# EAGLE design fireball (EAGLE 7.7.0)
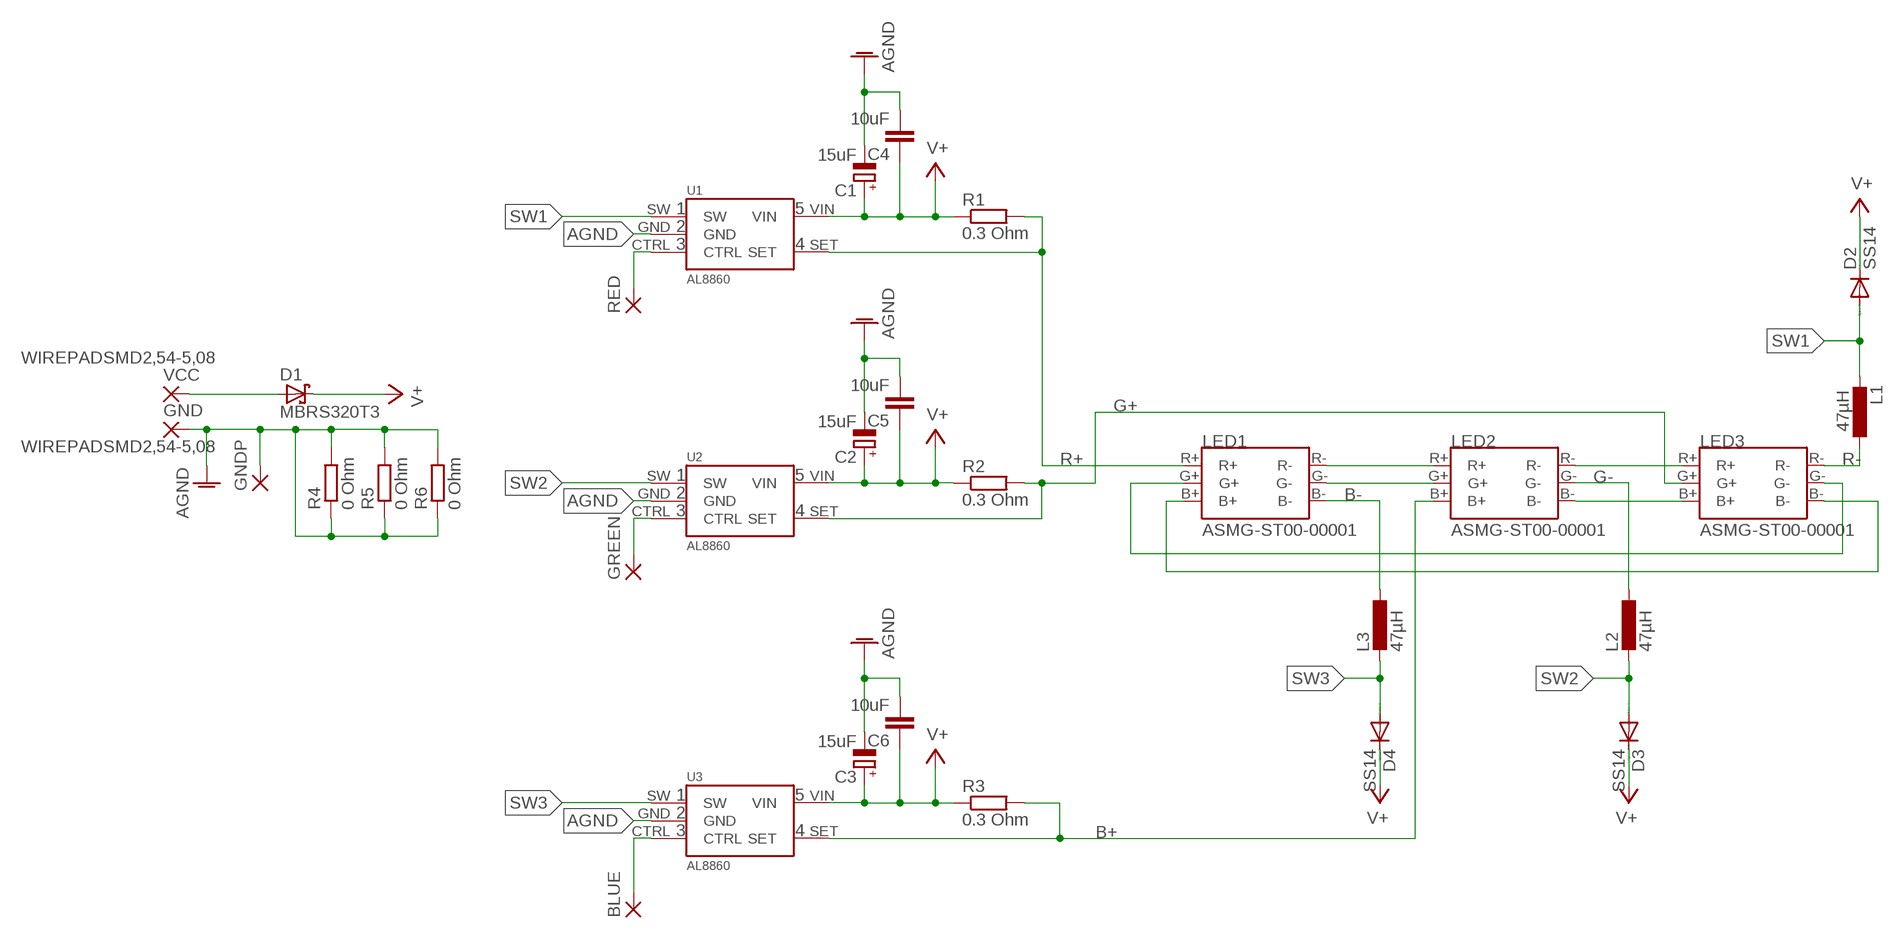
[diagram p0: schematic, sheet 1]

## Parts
BLUE  SMD2  [SMD1,27-2,54]
C1  15uF  CPOL-EUD/7343-31R  [D/7343-31R]
C2  15uF  CPOL-EUD/7343-31R  [D/7343-31R]
C3  15uF  CPOL-EUD/7343-31R  [D/7343-31R]
C4  10uF  C-EUC0805  [C0805]
C5  10uF  C-EUC0805  [C0805]
C6  10uF  C-EUC0805  [C0805]
D1  MBRS320T3  [SMC]
D2  SS14  DIODE-DO-214AC  [DO-214AC]
D3  SS14  DIODE-DO-214AC  [DO-214AC]
D4  SS14  DIODE-DO-214AC  [DO-214AC]
GND  WIREPADSMD2,54-5,08  [SMD2,54-5,08]
GNDP  SMD2  [SMD1,27-2,54]
GREEN  SMD2  [SMD1,27-2,54]
L1  47µH  L-EUL5038P  [L5038P]
L2  47µH  L-EUL5038P  [L5038P]
L3  47µH  L-EUL5038P  [L5038P]
LED1  ASMG-ST00-00001  [SMD]
LED2  ASMG-ST00-00001  [SMD]
LED3  ASMG-ST00-00001  [SMD]
R1  0.3 Ohm  R-EU_R1210  [R1210]
R2  0.3 Ohm  R-EU_R1210  [R1210]
R3  0.3 Ohm  R-EU_R1210  [R1210]
R4  0 Ohm  R-EU_R1206  [R1206]
R5  0 Ohm  R-EU_R1206  [R1206]
R6  0 Ohm  R-EU_R1206  [R1206]
RED  SMD2  [SMD1,27-2,54]
U1  AL8860  [TSOT-25-5]
U2  AL8860  [TSOT-25-5]
U3  AL8860  [TSOT-25-5]
VCC  WIREPADSMD2,54-5,08  [SMD2,54-5,08]

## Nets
AGND: C1.- C2.- C3.- C4.2 C5.2 C6.2 GND.1(P) GNDP.1(P) R4.1 R4.2 R5.1 R5.2 R6.1 R6.2 U1.GND U2.GND U3.GND
B+: LED2.B+ R3.2 U3.SET
B-: L3.1 LED1.B-
G+: LED3.G+ R2.2 U2.SET
G-: L2.1 LED2.G-
N$2: LED2.B- LED3.B+
N$3: LED1.B+ LED3.B-
N$6: LED1.G- LED2.G+
N$7: LED1.G+ LED3.G-
N$11: LED1.R- LED2.R+
N$12: LED2.R- LED3.R+
N$13: GREEN.1(P) U2.CTRL
N$14: BLUE.1(P) U3.CTRL
N$15: RED.1(P) U1.CTRL
N$16: D1.A VCC.1(P)
R+: LED1.R+ R1.2 U1.SET
R-: L1.1 LED3.R-
SW1: D2.A L1.2 U1.SW
SW2: D3.A L2.2 U2.SW
SW3: D4.A L3.2 U3.SW
V+: C1.+ C2.+ C3.+ C4.1 C5.1 C6.1 D1.C D2.C D3.C D4.C R1.1 R2.1 R3.1 U1.VIN U2.VIN U3.VIN

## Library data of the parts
BLUE GNDP GREEN RED = wirepad:SMD2: SMD PAD
C1-C3 = rcl:CPOL-EU: POLARIZED CAPACITOR, European symbol
C4-C6 = rcl:C-EU: CAPACITOR, European symbol
D1 = diode:MBRS3*0T3: SCHOTTKY BARRIER RECTIFIER 3.0 AMPERES 20, 30, 40 VOLT
D2-D4 = diode:DIODE-: DIODE
GND VCC = wirepad:WIREPAD: Wire PAD connect wire on PCB
L1-L3 = rcl:L-EU: INDUCTOR, European symbol
LED1-LED3 = broadcom:ASMG-ST00-00001
R1-R6 = rcl:R-EU_: RESISTOR, European symbol
U1-U3 = AL8860WT:AL8860

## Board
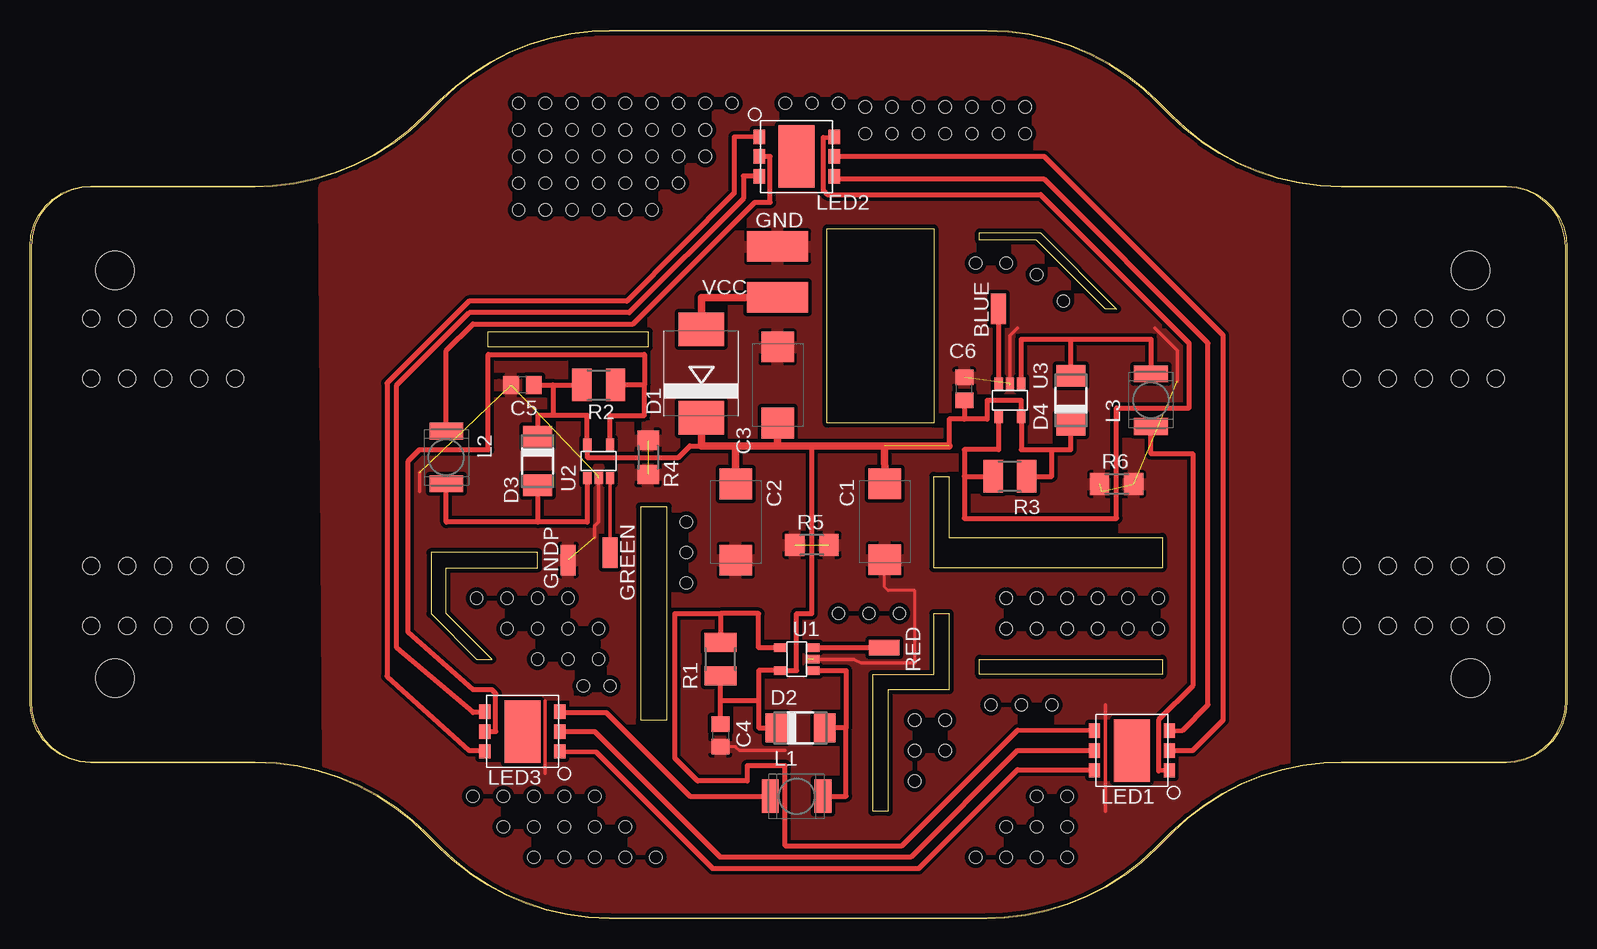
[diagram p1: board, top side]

Size 128.1 x 74.1 mm. Coordinates in mm from the lower left corner, seen from the top.
Outline: 551 segments
Copper layers (1*16): Top 0.035559375mm / dielectric 1.6mm / Bottom 0.035559375mm
Design rules "oshpark-2layer": minimum track width 6mil, minimum drill 10mil, track to track 6mil, track to pad 6mil, pad to pad 6mil, via to via 6mil, smd to smd 6mil, copper to edge 15mil, drill to drill 6mil, minimum pad ring 5mil, minimum via ring 5mil, stop-mask expansion 2.5mil, vias tented up to drill 0mil, thermal gap 10mil
Holes 3.2 mm at 120.09,20.05 120.09,54.05 7.09,54.05 7.09,20.05
Holes 1 mm at 42.32,21.64 44.86,21.64 47.4,21.64 47.4,24.18 44.86,26.72 44.86,24.18 42.32,24.18 42.32,26.72 39.78,26.72 39.78,24.18 37.24,26.72 83.91,26.72 86.45,26.72 88.99,26.72 91.53,26.72 83.91,24.18 86.45,24.18 88.99,24.18 91.53,24.18 81.37,26.72 81.37,24.18 94.07,26.72 94.07,24.18 73.75,16.56 76.29,16.56 73.75,14.02 76.29,14.02 73.75,11.48 83.91,10.21 86.45,10.21 86.45,7.67 83.91,7.67 81.37,7.67 78.83,5.13 81.37,5.13 83.91,5.13 86.45,5.13 67.4,25.45 69.94,25.45 72.48,25.45 54.7,33.07 54.7,30.53 54.7,27.99 47.08,10.21 44.54,10.21 44.54,7.67 42,10.21 39.46,10.21 36.92,10.21 39.46,7.67 42,7.67 47.08,7.67 47.08,5.13 44.54,5.13 42,5.13 49.62,5.13 49.62,7.67 52.16,5.13 78.83,54.66 81.37,54.66 83.91,53.71 86.14,51.48 80.1,17.83 82.64,17.83 85.18,17.83 69.62,65.45 71.85,65.45 74.07,65.45 76.29,65.45 78.52,65.45 80.74,65.45 82.96,65.45 69.62,67.68 71.85,67.68 74.07,67.68 76.29,67.68 78.52,67.68 80.74,67.68 82.96,67.68 58.51,67.99 62.96,67.99 67.4,67.99 65.18,67.99 46.13,19.42 48.35,19.42 56.29,67.99 54.07,67.99 51.84,67.99 49.62,67.99 56.29,65.77 56.29,63.55 54.07,65.77 54.07,63.55 51.84,61.33 51.84,63.55 51.84,65.77 49.62,65.77 49.62,63.55 49.62,61.33 47.4,67.99 45.18,67.99 42.95,67.99 40.73,67.99 40.73,65.77 42.95,65.77 45.18,65.77 47.4,65.77 47.4,63.55 45.18,63.55 42.95,63.55 40.73,63.55 40.73,61.33 42.95,61.33 45.18,61.33 47.4,61.33 40.73,59.1 42.95,59.1 45.18,59.1 47.4,59.1 49.62,59.1 51.84,59.1 54.07,61.33
Holes 1.4 mm at 5.09,50.05 8.09,50.05 11.09,50.05 14.09,50.05 17.09,50.05 5.09,45.05 8.09,45.05 11.09,45.05 14.09,45.05 17.09,45.05 5.09,29.41 8.09,29.41 11.09,29.41 14.09,29.41 17.09,29.41 5.09,24.41 8.09,24.41 11.09,24.41 14.09,24.41 17.09,24.41 110.19,50.05 113.19,50.05 116.19,50.05 119.19,50.05 122.19,50.05 110.19,45.05 113.19,45.05 116.19,45.05 119.19,45.05 122.19,45.05 110.19,29.41 113.19,29.41 116.19,29.41 119.19,29.41 122.19,29.41 110.19,24.41 113.19,24.41 116.19,24.41 119.19,24.41 122.19,24.41

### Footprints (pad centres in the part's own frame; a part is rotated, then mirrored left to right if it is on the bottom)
SMD1,27-2,54 = smd 1.27 x 2.54: 1 0,0
D/7343-31R = smd 2.55 x 2.7: + 3.175,0; - -3.175,0
C0805 = smd 1.3 x 1.5: 1 -0.95,0; 2 0.95,0
SMC = smd 2.8 x 3.8: A 3.7,0; C -3.7,0
DO-214AC = smd 1.8 x 2.4: A 2.025,0; C -2.025,0
SMD2,54-5,08 = smd 2.54 x 5.08: 1 0,0
L5038P = smd 1.4 x 2.8: 1 -2.2,0; 2 2.2,0
SMD = smd 0.95 x 1.2: B+ -3.125,-1.65; B- 3.125,-1.65; G+ -3.125,0; G- 3.125,0; R+ -3.125,1.65; R- 3.125,1.65 | smd 3 x 5.2: NC 0,0
R1210 = smd 1.6 x 2.7: 1 -1.4,0; 2 1.4,0
R1206 = smd 1.6 x 1.803: 1 -1.422,0; 2 1.422,0
TSOT-25-5 = smd 1 x 0.7: CTRL -1.4,-0.95; GND -1.4,0; SET 1.4,-0.95; SW -1.4,0.95; VIN 1.4,0.95

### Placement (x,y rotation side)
BLUE  80.74,50.85 0 top
C1  71.25,33.09 90 top
C2  58.83,33.07 90 top
C3  62.32,44.5 270 top
C4  57.56,15.29 270 top
C5  41.05,44.5 180 top
C6  77.88,44.18 90 top
D1  55.97,45.45 90 top
D2  64.23,15.93 0 top
D3  42.32,38.15 270 top
D4  86.77,43.23 90 top
GND  62.31,56.05 90 top
GNDP  44.86,29.89 0 top
GREEN  48.35,30.53 180 top
L1  63.91,10.21 0 top
L2  34.7,38.47 270 top
L3  93.44,43.23 90 top
LED1  91.85,14.02 0 top
LED2  63.91,63.55 180 top
LED3  41.05,15.61 0 top
R1  57.56,21.64 90 top
R2  47.4,44.5 0 top
R3  81.69,36.88 180 top
R4  51.53,38.47 90 top
R5  65.18,31.16 0 top
R6  90.58,36.24 0 top
RED  71.21,22.59 90 top
U1  63.91,21.64 180 top
U2  47.4,38.15 90 top
U3  81.69,43.23 270 top
VCC  62.32,51.8 270 top

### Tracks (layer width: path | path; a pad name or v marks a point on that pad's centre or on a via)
AGND  (12 unrouted)
  Top 0.254: 59.15,14.02 58.83,14.34 C4.2 | 68.67,21.64 69.31,21.32 | 73.75,21.32 73.75,27.36 71.53,27.36 71.21,27.67 71.21,30.21
  Top 0.305: 89.63,17.83 89.63,8.94 | 42.95,18.15 42.95,12.12 | 81.69,44.5 81.69,48.63 82.33,49.26 | 64.86,21.64 68.67,21.64 | 62.96,14.02 59.15,14.02 | 69.31,21.32 73.75,21.32 | 47.4,36.88 47.4,33.07 47.08,32.75 47.08,31.8 | 32.48,37.2 32.48,35.61 | 93.75,49.26 95.66,47.36 95.66,44.82
  Top 0.406: 89.31,35.61 89.31,36.88
  pour Top (isolate 0.305): 42.32,73.71 85.5,73.71 104.55,61.01 104.55,12.75 86.77,0.05 42.32,0.05 24.86,12.75 24.54,61.01
B+
  Top 0.406: U3.SET 80.74,39.1 77.88,39.1 77.88,36.88 | 77.88,36.88 77.88,33.39 90.58,33.39 90.58,42.59 96.61,42.59 96.61,47.99 84.23,60.38 66.45,60.38 66.13,60.69 66.13,65.14 LED2.B+ | 77.88,36.88 R3.2
B-
  Top 0.406: L3.1 93.44,38.78 96.93,38.78 96.93,19.42 94.07,16.56 94.07,12.32 LED1.B-
G+
  Top 0.406: U2.SET 48.35,40.69 48.35,41.96 51.21,41.96 51.21,44.5 | LED3.G+ 38.83,15.61 38.83,18.78 38.51,19.1 36.92,19.1 31.53,23.86 31.53,38.15 32.48,39.1 38.19,39.1 38.19,47.04 51.21,47.04 51.21,44.5 | 51.21,44.5 R2.2
G-
  Top 0.406: LED2.G- 61.69,63.55 61.69,59.74 60.42,59.74 50.26,49.58 36.92,49.58 34.7,47.36 L2.1
N$2
  Top 0.406: 37.8,14.02 LED3.B+ 37.69,14.02 36.61,14.02 29.76,20.21 29.76,44.65 36.59,51.48 49.76,51.48 58.69,60.49 58.69,65.17 LED2.B-
N$3
  Top 0.406: LED1.B+ 88.6,12.43 82.33,12.43 74.07,4.18 56.93,4.18 47.19,13.91 LED3.B-
N$6
  Top 0.406: LED1.G- 96.93,14.02 99.47,16.56 99.47,48.63 84.55,63.55 LED2.G+
N$7
  Top 0.406: LED1.G+ 82.33,14.02 73.44,5.13 57.56,5.13 47.08,15.61 LED3.G-
N$11
  Top 0.406: LED1.R- 96.09,15.72 98.2,17.83 98.2,47.99 84.55,61.64 67.36,61.64 LED2.R+
N$12
  Top 0.406: LED3.R+ 37.8,17.2 36.92,17.2 30.57,22.59 30.57,44.5 36.61,50.53 49.94,50.53 59.47,60.06 59.47,61.93 LED2.R-
N$13
  Top 0.305: GREEN.1 U2.CTRL
  Top 0.406: U2.CTRL
N$14
  Top 0.406: BLUE.1 80.74,48.31 U3.CTRL
N$15
  Top 0.406: RED.1 68.36,22.59 U1.CTRL
N$16
  Top 0.61: VCC.1 55.97,51.8 D1.A
R+
  Top 0.406: 57.56,25.45 R1.2 | U1.SET 60.73,22.59 60.73,25.45 57.56,25.45 | LED1.R+ 82.33,15.72 72.69,6.08 62.96,6.08 62.96,12.75 59.78,12.75 59.78,11.48 55.65,11.48 53.75,13.39 53.75,25.45 57.56,25.45
R-
  Top 0.406: LED3.R- 44.3,17.2 48.04,17.2 55.02,10.21 L1.1
SW1
  Top 0.406: U1.SW 68.04,20.69 68.04,15.93 | 68.04,15.93 D2.A | L1.2 68.04,10.21 68.04,15.93
SW2
  Top 0.406: U2.SW 46.45,33.07 42.32,33.07 | D3.A 42.32,33.07 | 42.32,33.07 34.7,33.07 L2.2
SW3
  Top 0.406: U3.SW 82.64,48.31 86.77,48.31 | 86.77,48.31 93.44,48.31 L3.2 | D4.A 86.77,48.31
V+  (1 unrouted)
  Top 0.2: U2.VIN 46.45,39.1
  Top 0.406: 60.73,18.15 60.73,20.69 U1.VIN 63.91,20.69 63.91,25.45 65.18,25.45 65.18,39.42 | 60.73,18.15 57.56,18.15 | 57.56,18.15 R1.1 | 60.73,18.15 60.73,15.93 D2.C | 43.59,44.5 R2.1 | U2.VIN 46.45,41.96 43.59,41.96 | 43.59,41.96 42.32,41.96 D3.C | C5.1 43.59,44.5 | 43.59,44.5 43.59,41.96 | U3.VIN 82.64,39.1 85.18,39.1 | 85.18,39.1 86.77,39.1 D4.C | 85.18,39.1 85.18,36.88 R3.1 | C4.1 57.56,18.15 | U3.VIN | U3.VIN 82.64,43.23 79.78,43.23 79.78,41.64 77.88,41.64 | 46.45,39.1 46.45,38.47 54.07,38.47 55.02,39.42 55.97,39.42 | 77.88,41.64 76.61,41.64 76.61,39.42 | C6.1 77.88,41.64
  Top 0.61: 58.83,39.42 C2.+ | C3.+ 62.32,39.42 | 62.32,39.42 58.83,39.42 | 58.83,39.42 55.97,39.42 D1.C | 62.32,39.42 65.18,39.42 65.81,39.42 76.61,39.42 | C1.+ 71.21,39.42

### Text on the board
200bmp: Fireball rev. F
